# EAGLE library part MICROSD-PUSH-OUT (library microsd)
T-Flash Push-Out Micro SD Card Reader 14.75mm x 14.5mm SMD with external pins
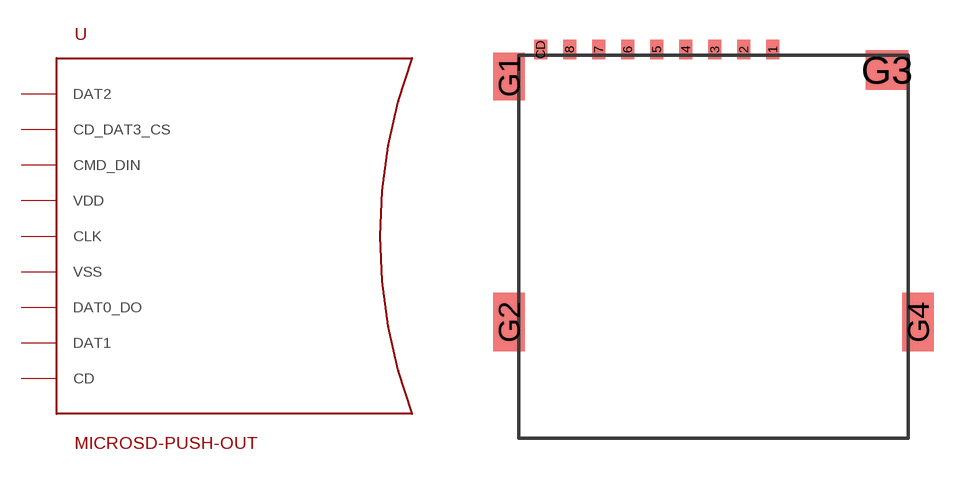
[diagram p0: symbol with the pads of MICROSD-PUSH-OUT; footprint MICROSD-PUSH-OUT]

Designator prefix -

## MICROSD-PUSH-OUT  [MICROSD-PUSH-OUT]
1  DAT2
2  CD_DAT3_CS
3  CMD_DIN
4  VDD
5  CLK
6  VSS
7  DAT0_DO
8  DAT1
CD  CD
G1  VSS
G2  VSS
G3  VSS
G4  VSS

## Footprint MICROSD-PUSH-OUT (pad centres in mm)
T-Flash Push-Out Micro SD Card Reader 9 pin SD mode and 7 pin SPI mode compatible 14.75mm x 14.5mm
smd 0.5 x 0.75: 1 9.625,0.225; 2 8.525,0.225; 3 7.425,0.225; 4 6.325,0.225; 5 5.225,0.225; 6 4.125,0.225; 7 3.025,0.225; 8 1.925,0.225; CD 0.825,0.225
smd 1.2 x 1.8: G1 -0.375,-0.8
smd 1.2 x 2.2: G2 -0.375,-10.1; G4 15.125,-10.1
smd 1.6 x 1.5: G3 13.95,-0.55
